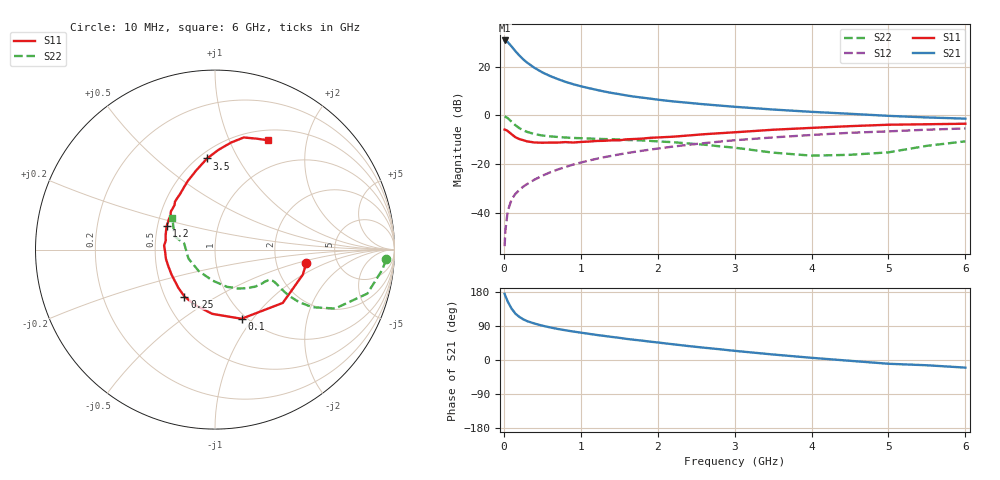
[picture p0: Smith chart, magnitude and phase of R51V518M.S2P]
! SIEMENS Small Signal Semiconductors
! BFR183
! Si NPN RF Bipolar Junction Transistor in SOT23
! VCE = 1.5 V  IC = 18 mA
! Common Emitter S-Parameters:  May  1996
# GHz  S  MA  R  50
!  f  S11  S21  S12  S22
! GHz  MAG  ANG  MAG  ANG  MAG  ANG  MAG  ANG
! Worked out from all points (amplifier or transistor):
!   36 points, 10 MHz to 6 GHz, reference 50 ohm
!   highest |S21| = 30.7 dB at 10 MHz (marker M1)
!   |S21| within 3 dB of that: start of sweep to 114.5 MHz
!   unconditionally stable (mu >= 1): 498.6 MHz to 2.457 GHz
!   at 250 MHz: K = 0.80, MSG = 26.1 dB, |S12| = -29.2 dB
!   at 1.4 GHz: K = 1.06, MAG = 11.4 dB, |S12| = -16.6 dB
!   at 6 GHz: K = 0.92, MSG = 2.0 dB, |S12| = -5.3 dB
!   S11 on the Smith chart (normalised r, x): 10 MHz: 2.98, -0.60; 100 MHz: 0.95, -0.88; 250 MHz: 0.63, -0.36; 1.2 GHz: 0.56, +0.16; 3.5 GHz: 0.55, +0.75; 6 GHz: 0.62, +1.40
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0.01  0.514 -8.3  34.35 174.6  0.0021 89.7  0.9547 -3.3
0.02  0.509 -15.9  34.21 169.0  0.0044 82.9  0.9394 -6.8
0.05  0.4804 -38.2  31.9 154.5  0.0109 74.3  0.8835 -16.1
0.1  0.4127 -69.0  25.94 135.8  0.019 69.3  0.7459 -26.1
0.15  0.3582 -92.5  20.79 122.4  0.0248 65.8  0.6308 -30.6
0.2  0.3286 -109.4  17.02 114.0  0.0295 65.6  0.5515 -32.0
0.25  0.3122 -123.0  14.18 107.6  0.0346 66.0  0.4981 -32.0
0.3  0.2947 -134.0  12.16 102.8  0.0391 67.2  0.4617 -31.5
0.4  0.2793 -150.3  9.416 96.1  0.0486 68.5  0.415 -30.1
0.5  0.2761 -161.2  7.625 90.6  0.0582 69.5  0.3878 -28.9
0.6  0.2782 -169.5  6.432 86.1  0.0681 69.4  0.3731 -28.5
0.7  0.2782 -177.7  5.567 82.0  0.078 69.8  0.3624 -28.4
0.8  0.2844 175.5  4.884 78.5  0.0876 69.3  0.353 -28.7
0.9  0.2789 169.8  4.371 75.2  0.0985 69.2  0.3462 -29.0
1.1  0.2914 159.4  3.639 69.3  0.1185 68.0  0.3371 -31.2
1.2  0.2998 154.1  3.356 66.3  0.1289 67.3  0.332 -32.1
1.6  0.3249 139.2  2.559 55.6  0.1693 63.6  0.3142 -38.0
2.2  0.3668 121.8  1.939 41.5  0.2305 57.1  0.2831 -49.5
3.5  0.5095 95.0  1.321 14.5  0.3547 40.1  0.173 -94.5
4.5  0.6035 81.4  1.081 -2.1  0.4413 26.9  0.1561 -161.4
5.5  0.66 69.5  0.91 -13.9  0.5108 15.0  0.2386 161.8
6  0.6765 64.3  0.86 -20.1  0.5414 7.3  0.295 143.5
